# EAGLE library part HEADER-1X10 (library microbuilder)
PIN HEADER
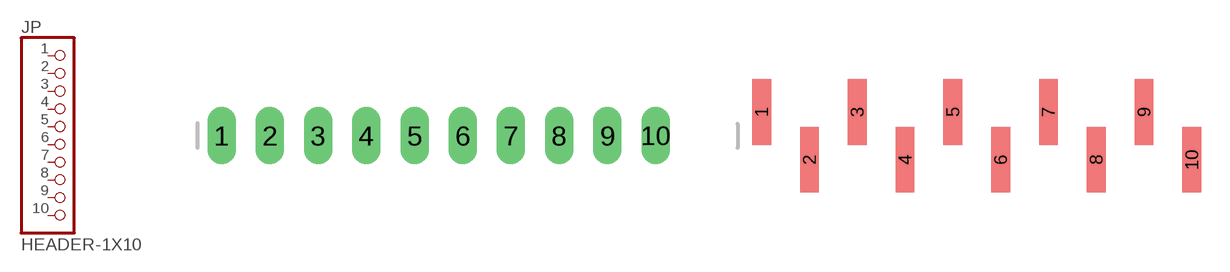
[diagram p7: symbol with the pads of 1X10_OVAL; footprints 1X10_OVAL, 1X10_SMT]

Designator prefix JP

## HEADER-1X10  [1X10_OVAL]
1  1  pas
2  2  pas
3  3  pas
4  4  pas
5  5  pas
6  6  pas
7  7  pas
8  8  pas
9  9  pas
10  10  pas

## HEADER-1X10SMT  [1X10_SMT]
Pads as for 1X10_OVAL

## HEADER-1X10ROUND  [1X10_ROUND]
Pads as for 1X10_OVAL

## HEADER-1X101X10_2MM  [1X10_ROUND_2MM]
Pads as for 1X10_OVAL

## HEADER-1X10THICKER  [1X10_ROUND_76]
Pads as for 1X10_OVAL

## HEADER-1X1070MIL  [1X10_ROUND70]
Pads as for 1X10_OVAL

## Footprint 1X10_OVAL (pad centres in mm)
1x10 PIN HEADER
drill 1 long: 1 -11.43,0; 2 -8.89,0; 3 -6.35,0; 4 -3.81,0; 5 -1.27,0; 6 1.27,0; 7 3.81,0; 8 6.35,0; 9 8.89,0; 10 11.43,0

## Footprint 1X10_SMT (pad centres in mm)
Pin Headers 10 Pin, 0.1"/2.54mm pitch, SMT
smd 1 x 3.5: 1 -11.43,1.27; 2 -8.89,-1.27; 3 -6.35,1.27; 4 -3.81,-1.27; 5 -1.27,1.27; 6 1.27,-1.27; 7 3.81,1.27; 8 6.35,-1.27; 9 8.89,1.27; 10 11.43,-1.27

## Footprint 1X10_ROUND (pad centres in mm)
drill 1 pad 1.676: 1 -11.43,0; 2 -8.89,0; 3 -6.35,0; 4 -3.81,0; 5 -1.27,0; 6 1.27,0; 7 3.81,0; 8 6.35,0; 9 8.89,0; 10 11.43,0

## Footprint 1X10_ROUND_2MM (pad centres in mm)
1x10 2.0mm Header Pins
drill 1 pad 1.5: 1 -10,0; 2 -8,0; 3 -6,0; 4 -4,0; 5 -2,0; 6 0,0; 7 2,0; 8 4,0; 9 6,0; 10 8,0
